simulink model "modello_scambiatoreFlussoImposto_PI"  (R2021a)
settings: Solver=FixedStepAuto  StartTime=0.0  StopTime=3000  FixedStep=0.01  RelTol=1e-3
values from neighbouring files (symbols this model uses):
  Ki = 2287    [scambiatoredicalore_dati.m]    (also in scambiatoremodelloTD.m)
undefined symbols (not defined in the file or in its folder): c, delta, deltaTi, Kp, m, Qeq, Qfin, T0eq, Tieq, weq
libraries: pid_lib x1

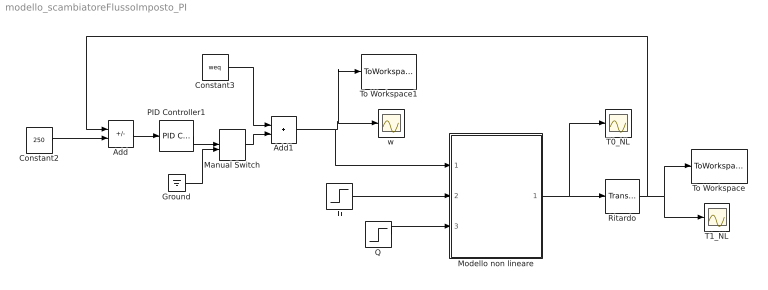
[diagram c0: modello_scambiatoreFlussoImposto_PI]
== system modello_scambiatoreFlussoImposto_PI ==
  Add : Sum  Inputs=+-
  Add1 : Sum
  Constant2 : Constant  Value=250
  Constant3 : Constant  Value=weq
  Ground : Ground
  Manual Switch : ManualSwitch
  Modello non lineare : Subsystem
  PID Controller1 : pid_lib/PID Controller  Controller=PID  Form=Parallel  TimeDomain=Continuous-time  UseExternalTs=off  SampleTime=-1  IntegratorMethod=Forward Euler  FilterMethod=Forward Euler  ControllerParametersSource=internal  P=Kp  I=Ki  D=0  UseFilter=on  N=100  TunerSelectOption=Transfer Function Based (PID Tuner App)  InitialConditionSource=internal  InitialConditionForIntegrator=0  InitialConditionForFilter=0  DifferentiatorICPrevScaledInput=0  ExternalReset=none  TrackingMode=off  Kt=1  LimitOutput=off  SatLimitsSource=internal  UpperSaturationLimit=inf  LowerSaturationLimit=-inf  LinearizeAsGain=on  AntiWindupMode=none  Kb=1  POutMin=[]  POutMax=[]  IOutMin=[]  IOutMax=[]  DOutMin=[]  DOutMax=[]  NOutMin=[]  NOutMax=[]  SumOutMin=[]  SumOutMax=[]  SaturationOutMin=[]  SaturationOutMax=[]  PParamMin=[]  PParamMax=[]  IParamMin=[]  IParamMax=[]  DParamMin=[]  DParamMax=[]  NParamMin=[]  NParamMax=[]  KbParamMin=[]  KbParamMax=[]  KtParamMin=[]  KtParamMax=[]  KbOutMin=[]  KbOutMax=[]  KtOutMin=[]  KtOutMax=[]  IntegratorOutMin=[]  IntegratorOutMax=[]  FilterOutMin=[]  FilterOutMax=[]  SumI1OutMin=[]  SumI1OutMax=[]  SumI2OutMin=[]  SumI2OutMax=[]  SumI3OutMin=[]  SumI3OutMax=[]  SumI4OutMin=[]  SumI4OutMax=[]  SumDOutMin=[]  SumDOutMax=[]  DifferentiatorOutMin=[]  DifferentiatorOutMax=[]  FilterDiffOutCoefMin=[]  FilterDiffOutCoefMax=[]  ReciprocalOutMin=[]  ReciprocalOutMax=[]  SumDenOutMin=[]  SumDenOutMax=[]  SumNumOutMin=[]  SumNumOutMax=[]  DivideOutMin=[]  DivideOutMax=[]  UdiffTsProdOutMin=[]  UdiffTsProdOutMax=[]  NTsProdOutMin=[]  NTsProdOutMax=[]  UintegralTsProdOutMin=[]  UintegralTsProdOutMax=[]  UngainTsProdOutMin=[]  UngainTsProdOutMax=[]  IntegratorContinuousStateAttributes=''  IntegratorStateMustResolveToSignalObject=off  IntegratorRTWStateStorageClass=Auto  FilterContinuousStateAttributes=''  FilterStateMustResolveToSignalObject=off  FilterRTWStateStorageClass=Auto  ParallelPVariant=InternalParameters  IdealPVariant=Disabled  IVariant=InternalParameters  DVariant=InternalParameters  IntegratorVariant=Continuous  SatVariant=Disabled  AWVariant=Passthrough  PCopyVariant=Disabled  TRVariant=Disabled  FdbkBlocksVariant=Forward  IdealPFdbkVariant=Disabled  SatFdbkVariant=Disabled  DerivativeFilterVariant=ContFilter  NVariant=InternalParameters  NCopyVariant=Disabled  FilterICVariant=InternalICsFilter  IntegratorICVariant=InternalICs  ExternalResetVariant=Disabled  TRSumVariant=Passthrough  SumFdbkVariant=Disabled  SumVariant=Sum_PID  TsampFilterVariant=InternalTs  TsampNgainVariant=Passthrough  TsampIntegralVariant=Passthrough  ExternalSaturationOutDataTypeStr=Inherit: Same as second input
  Q : Step  Time=600  Before=Qeq  After=Qfin  SampleTime=0
  Ritardo : TransportDelay  DelayTime=delta  InitialOutput=T0eq  BufferSize=4000
  T0_NL : Scope
  T1_NL : Scope
  Ti : Step  Time=50  Before=Tieq  After=Tieq+deltaTi  SampleTime=0
  To Workspace : ToWorkspace  VariableName=T1NL  SaveFormat=Timeseries  SampleTime=-1
  To Workspace1 : ToWorkspace  VariableName=w  SaveFormat=Timeseries  SampleTime=-1
  w : Scope
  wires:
  Ti/1 -> Modello non lineare/2(Ti)
  Q/1 -> Modello non lineare/3(Q)
  Ritardo/1 -> To Workspace/1, T1_NL/1, Add/1
  Modello non lineare/1(T0) -> Ritardo/1, T0_NL/1
  Add1/1 -> Modello non lineare/1(w), To Workspace1/1, w/1
  Constant2/1 -> Add/2
  Add/1 -> PID Controller1/1
  Constant3/1 -> Add1/1
  PID Controller1/1 -> Manual Switch/1
  Manual Switch/1 -> Add1/2
  Ground/1 -> Manual Switch/2

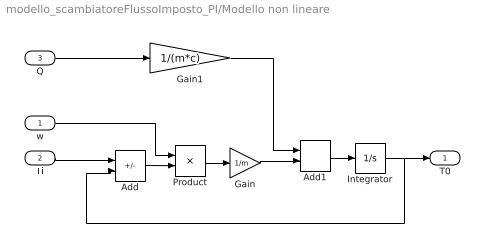
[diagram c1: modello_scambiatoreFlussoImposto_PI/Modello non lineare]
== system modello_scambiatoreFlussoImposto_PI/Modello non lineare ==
  w : Inport
  Ti : Inport  Port=2
  Q : Inport  Port=3
  Add : Sum  Inputs=+-
  Add1 : Sum
  Gain : Gain  Gain=1/m
  Gain1 : Gain  Gain=1/(m*c)
  Integrator : Integrator  InitialCondition=T0eq
  Product : Product
  T0 : Outport
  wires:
  Ti/1 -> Add/1
  Integrator/1 -> Add/2, T0/1
  Add/1 -> Product/2
  w/1 -> Product/1
  Product/1 -> Gain/1
  Gain/1 -> Add1/2
  Add1/1 -> Integrator/1
  Q/1 -> Gain1/1
  Gain1/1 -> Add1/1
